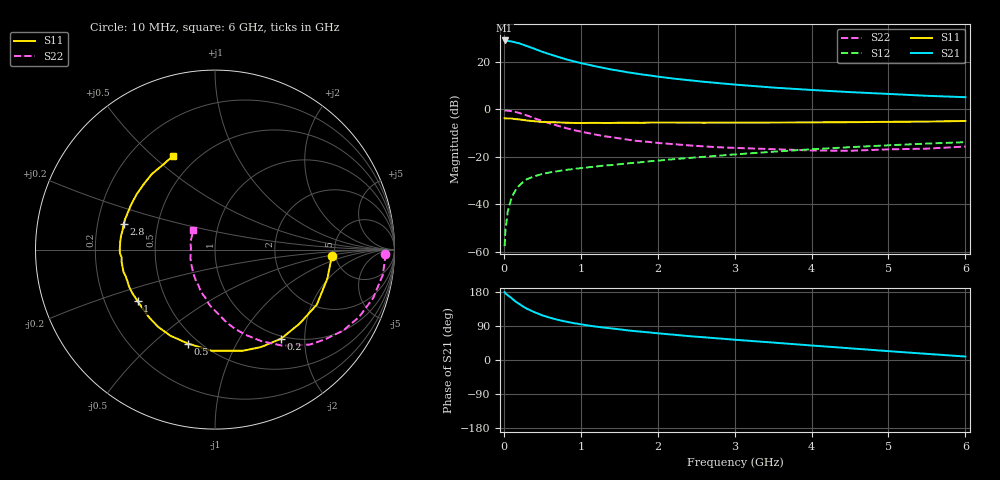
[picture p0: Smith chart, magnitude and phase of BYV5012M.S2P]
! SIEMENS Small Signal Semiconductors
! BFY420
! Si NPN RF SIEGET Grounded Emitter Transistor in MICRO-X
! VCE = 0.5 V  IC = 12 mA
! Common Emitter S-Parameters:  October  1996
# GHz  S  MA  R  50
!  f  S11  S21  S12  S22
! GHz  MAG  ANG  MAG  ANG  MAG  ANG  MAG  ANG
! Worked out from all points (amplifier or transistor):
!   36 points, 10 MHz to 6 GHz, reference 50 ohm
!   highest |S21| = 29.2 dB at 10 MHz (marker M1)
!   |S21| within 3 dB of that: start of sweep to 353.5 MHz
!   unconditionally stable (mu >= 1): 2.07 GHz to end of sweep
!   at 250 MHz: K = 0.23, MSG = 29.0 dB, |S12| = -30.6 dB
!   at 1.4 GHz: K = 0.85, MSG = 20.2 dB, |S12| = -23.5 dB
!   at 6 GHz: K = 1.13, MAG = 7.3 dB, |S12| = -13.8 dB
!   S11 on the Smith chart (normalised r, x): 10 MHz: 4.69, -0.62; 200 MHz: 0.96, -1.54; 500 MHz: 0.44, -0.65; 1 GHz: 0.34, -0.27; 2.8 GHz: 0.31, +0.12; 6 GHz: 0.37, +0.58
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0.01  0.6539 -3.3  28.68 179.1  0.0013 88.6  0.949 -1.4
0.02  0.6479 -6.2  28.59 176.0  0.0027 85.9  0.9486 -3.2
0.05  0.6467 -14.2  27.91 171.0  0.0069 85.4  0.9457 -8.5
0.1  0.6449 -28.3  27.33 163.3  0.0137 78.6  0.9218 -17.0
0.15  0.6264 -41.1  26.09 154.5  0.0196 70.9  0.886 -25.1
0.2  0.6181 -53.3  24.94 148.0  0.0248 67.4  0.8449 -32.3
0.25  0.6006 -64.7  23.36 141.1  0.0294 61.9  0.7916 -39.1
0.3  0.5849 -74.4  21.82 135.3  0.0337 58.7  0.7483 -45.0
0.4  0.5638 -92.1  19.07 126.0  0.0391 53.3  0.6521 -55.1
0.5  0.5446 -106.1  16.5 117.8  0.0435 49.1  0.5711 -63.2
0.6  0.5403 -117.4  14.61 111.6  0.047 47.0  0.5067 -70.0
0.7  0.5346 -126.5  13 106.1  0.0498 45.4  0.4542 -76.0
0.8  0.5263 -134.6  11.6 101.6  0.0527 43.5  0.4086 -81.2
1  0.5177 -146.4  9.557 94.2  0.0577 43.3  0.3412 -89.8
1.1  0.5205 -151.7  8.808 91.0  0.0602 43.1  0.317 -94.4
1.6  0.524 -170.0  6.132 78.4  0.0725 42.8  0.2324 -111.7
2.2  0.5299 175.6  4.503 66.9  0.0889 42.1  0.186 -128.9
2.8  0.5284 164.5  3.591 56.8  0.1062 40.2  0.1594 -144.6
3.5  0.5298 152.6  2.905 46.0  0.1282 36.6  0.1453 -160.4
4.5  0.5393 137.2  2.327 30.9  0.1602 28.6  0.1344 176.4
5.5  0.5552 121.1  1.946 16.2  0.1905 19.2  0.1491 149.3
6  0.5725 114.1  1.818 9.2  0.2044 14.3  0.165 138.3
